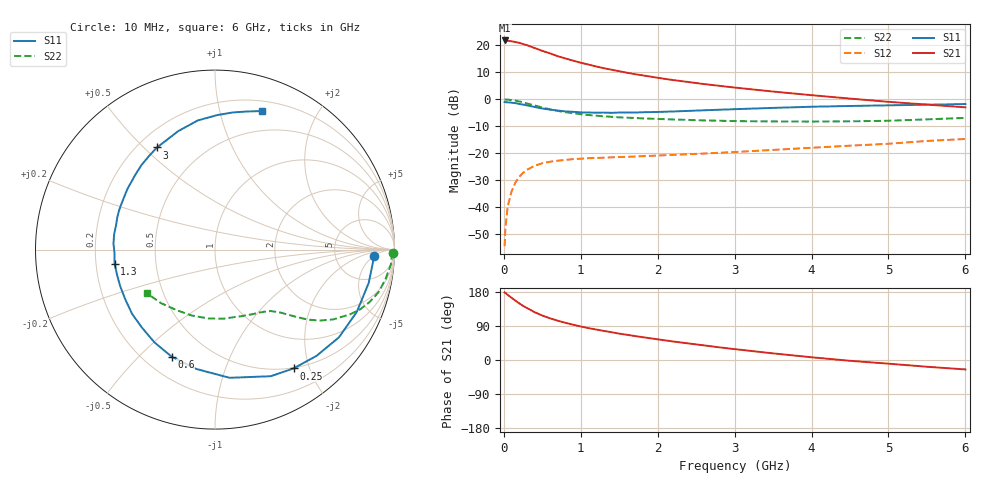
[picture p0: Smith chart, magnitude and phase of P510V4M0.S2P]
! SIEMENS Small Signal Semiconductors
! BFP183
! Si NPN RF Bipolar Junction Transistor in SOT143
! VCE = 10 V  IC = 4 mA
! Common Emitter S-Parameters:  March  1996
# GHz  S  MA  R  50
!  f  S11  S21  S12  S22
! GHz  MAG  ANG  MAG  ANG  MAG  ANG  MAG  ANG
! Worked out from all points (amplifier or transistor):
!   36 points, 10 MHz to 6 GHz, reference 50 ohm
!   highest |S21| = 21.8 dB at 10 MHz (marker M1)
!   |S21| within 3 dB of that: start of sweep to 420 MHz
!   unconditionally stable (mu >= 1): 1.808 GHz to 5.804 GHz
!   at 250 MHz: K = 0.18, MSG = 23.9 dB, |S12| = -27.3 dB
!   at 1.4 GHz: K = 0.84, MSG = 16.2 dB, |S12| = -21.5 dB
!   at 6 GHz: K = 0.97, MSG = 5.9 dB, |S12| = -14.7 dB
!   S11 on the Smith chart (normalised r, x): 10 MHz: 15, -5; 250 MHz: 0.49, -1.76; 600 MHz: 0.31, -0.63; 1.3 GHz: 0.28, -0.06; 3 GHz: 0.28, +0.55; 6 GHz: 0.29, +1.35
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0.01  0.8853 -2.4  12.26 178.3  0.0019 79.9  0.9913 -1.0
0.02  0.8826 -4.7  12.23 177.1  0.004 81.1  0.9866 -2.0
0.05  0.8764 -12.2  12.08 171.9  0.0103 84.5  0.9831 -4.9
0.1  0.863 -23.7  11.84 164.2  0.0195 76.1  0.9639 -9.9
0.15  0.846 -35.3  11.45 156.7  0.0287 70.4  0.9416 -14.6
0.2  0.8189 -46.3  11.07 149.5  0.0366 65.4  0.9099 -18.7
0.25  0.7937 -56.5  10.54 142.8  0.0433 60.3  0.8744 -22.4
0.3  0.7709 -66.2  10.03 137.3  0.0493 55.7  0.8345 -25.6
0.4  0.7189 -83.5  8.894 126.2  0.0586 48.8  0.766 -30.5
0.5  0.6729 -99.1  7.861 117.3  0.0652 42.8  0.7037 -34.2
0.6  0.6434 -112.1  7.067 110.0  0.0696 38.3  0.6497 -36.9
0.7  0.6171 -123.2  6.268 103.7  0.0726 35.2  0.6081 -38.7
0.8  0.5955 -133.1  5.696 98.1  0.0752 32.8  0.5759 -40.2
1.1  0.5663 -158.8  4.384 84.1  0.0809 28.0  0.5101 -43.6
1.3  0.5649 -172.0  3.756 76.7  0.0827 26.4  0.4827 -45.8
1.7  0.5675 166.3  2.919 63.4  0.0869 25.2  0.4493 -50.5
2.2  0.5936 145.4  2.264 48.9  0.0931 25.5  0.4222 -57.4
3  0.6543 119.6  1.645 28.7  0.1052 26.5  0.3932 -72.1
3.5  0.6909 107.3  1.387 17.5  0.1152 26.7  0.388 -82.9
4.5  0.7494 89.1  1.028 -2.1  0.1379 24.7  0.3896 -109.5
5.5  0.7909 76.7  0.796 -17.8  0.1688 21.7  0.4236 -135.2
6  0.8149 71.3  0.708 -24.9  0.1836 18.2  0.4513 -147.5
